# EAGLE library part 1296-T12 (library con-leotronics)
1.27mm SINGLE ROW FEMALE SOCKET Source: http://www.leotronics.co.uk/Conexcon/Data%20Sheets/sec.%20A/1296ing.pdf
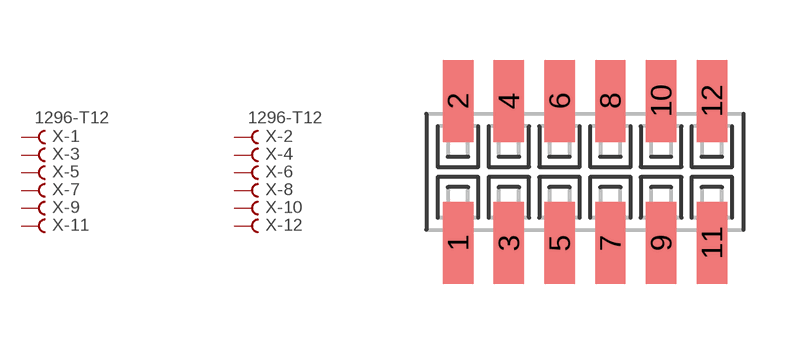
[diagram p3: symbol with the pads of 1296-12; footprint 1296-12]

Designator prefix X; gates -1=FVAL -2=FVAL -3=F -4=F -5=F -6=F -7=F -8=F -9=F -10=F -11=F -12=F

## 1296-T12 (OC_FARNELL: unknown; OC_NEWARK: unknown)  [1296-12]
1  -1:B  pas
2  -2:B  pas
3  -3:B  pas
4  -4:B  pas
5  -5:B  pas
6  -6:B  pas
7  -7:B  pas
8  -8:B  pas
9  -9:B  pas
10  -10:B  pas
11  -11:B  pas
12  -12:B  pas

## Footprint 1296-12 (pad centres in mm)
1.27mm SINGLE ROW FEMALE SOCKET Source: http://www.leotronics.co.uk/Conexcon/Data%20Sheets/sec.%20A/1296ing.pdf
smd 0.76 x 2.05: 1 -3.175,-1.78; 2 -3.175,1.78; 3 -1.905,-1.78; 4 -1.905,1.78; 5 -0.635,-1.78; 6 -0.635,1.78; 7 0.635,-1.78; 8 0.635,1.78; 9 1.905,-1.78; 10 1.905,1.78; 11 3.175,-1.78; 12 3.175,1.78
